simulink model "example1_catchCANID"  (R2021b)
settings: Solver=FixedStepAuto  StartTime=0.0  StopTime=inf  FixedStep=0.1  RelTol=1e-3
libraries: CANBusLib x2

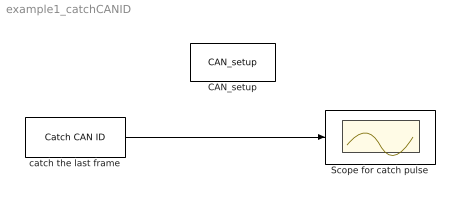
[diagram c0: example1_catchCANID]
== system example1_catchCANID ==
  CAN_setup : CANBusLib/CAN_setup  Priority=1  g1_cmbPortName="\"COM17\""  g2_cmbBaudRate=250000  g3_chkEcho=off  g59_chkTerminator=on  g4_cmbObjectID=0  g5_chkEnableSync=off  g10_chkRxWDEnable=off  g12_cmbRxWDLen=1  g13_cmbRxWDStartPos=1  g_60_cmbRxWDMode=0  g15_chkTxWDEnable=off  g17_cmbTxWDLen=1  g18_cmbTxWDStartPos=1  g_61_cmbTxWDMode=0  g20_ediF1=0  g21_chkExt4F1=off  g22_ediF2=0  g23_chkExt4F2=off  g24_ediF3=0  g25_chkExt4F3=off  g26_ediF4=0  g27_chkExt4F4=off  g28_ediF5=0  g29_chkExt4F5=off  g30_ediF6=0  g31_chkExt4F6=off  g32_ediF7=0  g33_chkExt4F7=off  g34_ediF8=0  g35_chkExt4F8=off  g36_ediM1=0  g37_ediF9=0  g38_chkExt4F9=on  g39_ediF10=0  g40_chkExt4F10=on  g41_ediF11=0  g42_chkExt4F11=on  g43_ediF12=0  g44_chkExt4F12=on  g45_ediM2=0  g46_ediF13=0  g47_chkExt4F13=off  g48_ediF14=0  g49_chkExt4F14=on  g50_ediF15=0  g51_chkExt4F15=on  g52_ediF16=0  g53_chkExt4F16=on  g54_ediM3=0  g62_autoFresh=on
  Scope for catch pulse : Scope
  catch the last frame : CANBusLib/Catch CAN ID  g1_ObjectID=0  g2_CANID=44  g3_Extended=off  g4_chkCatchLast=on  g5_lastFrameNo=2
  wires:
  catch the last frame/1 -> Scope for catch pulse/1
